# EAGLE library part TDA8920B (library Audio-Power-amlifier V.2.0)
The TDA8920B is a high efficiency class-D audio power amplifier with very low dissipation. The typical output power is 2 ´ 100 W. The device is available in the HSOP24 power package and in the DBS23P through-hole power package. The amplifier operates over a wide supply voltage range from ±12.5 V to ±30 V and consumes a very low quiescent current.
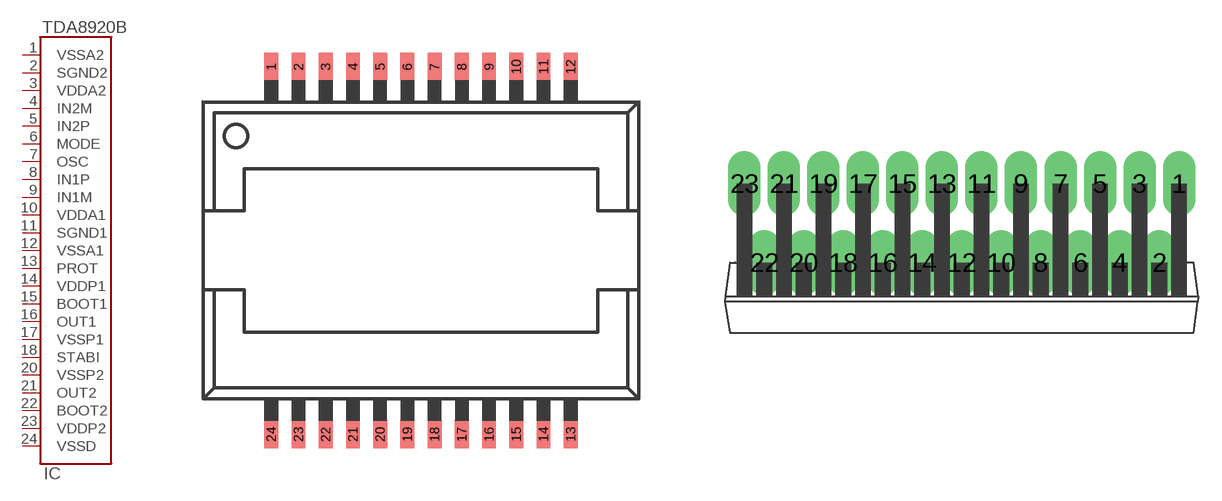
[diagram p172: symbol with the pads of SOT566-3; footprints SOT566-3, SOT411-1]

Designator prefix IC

## TDA8920BTDA8920BTH  [SOT566-3]
1  VSSA2  pwr
2  SGND2  pwr
3  VDDA2  pwr
4  IN2M  in
5  IN2P  in
6  MODE  in
7  OSC  in
8  IN1P  in
9  IN1M  in
10  VDDA1  pwr
11  SGND1  pwr
12  VSSA1  pwr
13  PROT
14  VDDP1  pwr
15  BOOT1
16  OUT1  out
17  VSSP1  pwr
18  STABI  pwr
20  VSSP2  pwr
21  OUT2  out
22  BOOT2
23  VDDP2  pwr
24  VSSD  pwr

## TDA8920BTDA8920BJ  [SOT411-1]
1  MODE  in
2  IN2P  in
3  IN2M  in
4  VDDA2  pwr
5  SGND2  pwr
6  VSSA2  pwr
7  VSSD  pwr
8  VDDP2  pwr
9  BOOT2
10  OUT2  out
11  VSSP2  pwr
12  STABI  pwr
13  VSSP1  pwr
14  OUT1  out
15  BOOT1
16  VDDP1  pwr
17  PROT
18  VSSA1  pwr
19  SGND1  pwr
20  VDDA1  pwr
21  IN1M  in
22  IN1P  in
23  OSC  in

## Footprint SOT566-3 (pad centres in mm)
smd 0.508 x 1.016: 1 -5.5,6.75; 2 -4.5,6.75; 3 -3.5,6.75; 4 -2.5,6.75; 5 -1.5,6.75; 6 -0.5,6.75; 7 0.5,6.75; 8 1.5,6.75; 9 2.5,6.75; 10 3.5,6.75; 11 4.5,6.75; 12 5.5,6.75; 13 5.5,-6.75; 14 4.5,-6.75; 15 3.5,-6.75; 16 2.5,-6.75; 17 1.5,-6.75; 18 0.5,-6.75; 19 -0.5,-6.75; 20 -1.5,-6.75; 21 -2.5,-6.75; 22 -3.5,-6.75; 23 -4.5,-6.75; 24 -5.5,-6.75

## Footprint SOT411-1 (pad centres in mm)
drill 1.4 long: 1 13.97,5.08; 2 12.7,0; 3 11.43,5.08; 4 10.16,0; 5 8.89,5.08; 6 7.62,0; 7 6.35,5.08; 8 5.08,0; 9 3.81,5.08; 10 2.54,0; 11 1.27,5.08; 12 0,0; 13 -1.27,5.08; 14 -2.54,0; 15 -3.81,5.08; 16 -5.08,0; 17 -6.35,5.08; 18 -7.62,0; 19 -8.89,5.08; 20 -10.16,0; 21 -11.43,5.08; 22 -12.7,0; 23 -13.97,5.08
